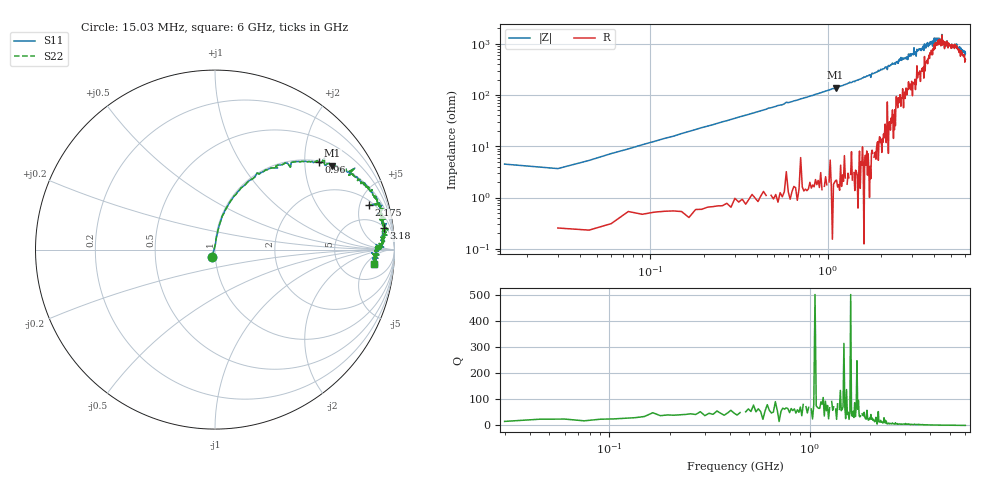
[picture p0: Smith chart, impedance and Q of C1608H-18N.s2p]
!	Network	Analyzer	HP8753E.07.74:	Oct	30	2002	Serial	No.	JP38451487
!	Hewlett-Packard
!	7	Sep	2009	10:20:29
!	Frequency	S11	S21	S12	S22
#	HZ	S	RI	R	50
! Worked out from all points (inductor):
!   400 points, 15.03 MHz to 6 GHz, reference 50 ohm
!   read as one part in series: L = 18.8 nH near 45.03 MHz
!   highest Q = 77.9 at 1.11 GHz (marker M1), where L = 19.8 nH
!   self-resonance near 4.603 GHz
!   S11 on the Smith chart (normalised r, x): 15.03 MHz: 0.96, -0.08; 960 MHz: 1.03, +2.34; 2.175 GHz: 2.47, +6.09; 3.18 GHz: 5, +13; 6 GHz: 11, -8
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1.502992e7  -0.0162 -0.042  1.02 0.042  1.02 0.042  -0.0162 -0.042
3.002985e7  0.00374 0.0364  0.996 -0.0364  0.996 -0.0364  0.00374 0.0364
7.502962e7  0.013 0.0871  0.987 -0.0871  0.987 -0.0871  0.013 0.0871
1.500292e8  0.0355 0.17  0.965 -0.17  0.965 -0.17  0.0355 0.17
3.150284e8  0.126 0.321  0.874 -0.321  0.874 -0.321  0.126 0.321
9.600252e8  0.577 0.487  0.423 -0.487  0.423 -0.487  0.577 0.487
1.020025e9  0.609 0.48  0.391 -0.48  0.391 -0.48  0.609 0.48
1.110024e9  0.654 0.468  0.346 -0.468  0.346 -0.468  0.654 0.468
2.01002e9  0.897 0.283  0.103 -0.283  0.103 -0.283  0.897 0.283
2.175019e9  0.859 0.248  0.141 -0.248  0.141 -0.248  0.859 0.248
3.015015e9  0.955 0.145  0.0454 -0.145  0.0454 -0.145  0.955 0.145
3.180014e9  0.942 0.121  0.0577 -0.121  0.0577 -0.121  0.942 0.121
3.91501e9  0.924 0.0695  0.0762 -0.0695  0.0762 -0.0695  0.924 0.0695
4.00501e9  0.943 0.0447  0.0574 -0.0447  0.0574 -0.0447  0.943 0.0447
4.365008e9  0.915 0.0343  0.0851 -0.0343  0.0851 -0.0343  0.915 0.0343
4.425008e9  0.94 0.0138  0.0604 -0.0138  0.0604 -0.0138  0.94 0.0138
4.455008e9  0.908 0.0205  0.0915 -0.0205  0.0915 -0.0205  0.908 0.0205
4.575007e9  0.897 0.0285  0.103 -0.0285  0.103 -0.0285  0.897 0.0285
4.725006e9  0.919 0.00269  0.0809 -0.00269  0.0809 -0.00269  0.919 0.00269
4.785006e9  0.894 0.0119  0.106 -0.0119  0.106 -0.0119  0.894 0.0119
5.010005e9  0.9 0.000824  0.0997 -0.000824  0.0997 -0.000824  0.9 0.000824
6e9  0.888 -0.0804  0.112 0.0804  0.112 0.0804  0.888 -0.0804
